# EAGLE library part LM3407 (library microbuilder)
LM3407 - 350 mA, Constant Current Output Floating Buck Switching Converter for High Power LEDs
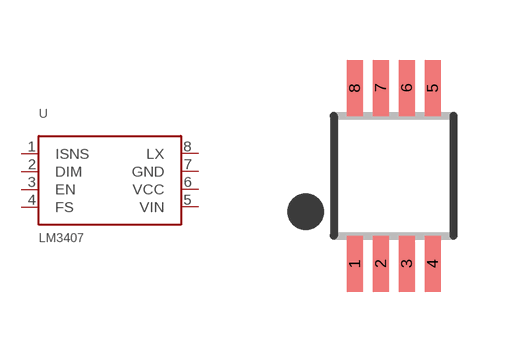
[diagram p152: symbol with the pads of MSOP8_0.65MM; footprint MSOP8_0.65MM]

Designator prefix U

## LM3407  [MSOP8_0.65MM]
1  ISNS
2  DIM
3  EN
4  FS
5  VIN
6  VCC
7  GND
8  LX

## Footprint MSOP8_0.65MM (pad centres in mm)
Source: http://www.intersil.com/data/fn/fn7833.pdf
smd 0.4 x 1.4: 1 -0.975,-2.2; 2 -0.325,-2.2; 3 0.325,-2.2; 4 0.975,-2.2; 5 0.975,2.2; 6 0.325,2.2; 7 -0.325,2.2; 8 -0.975,2.2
